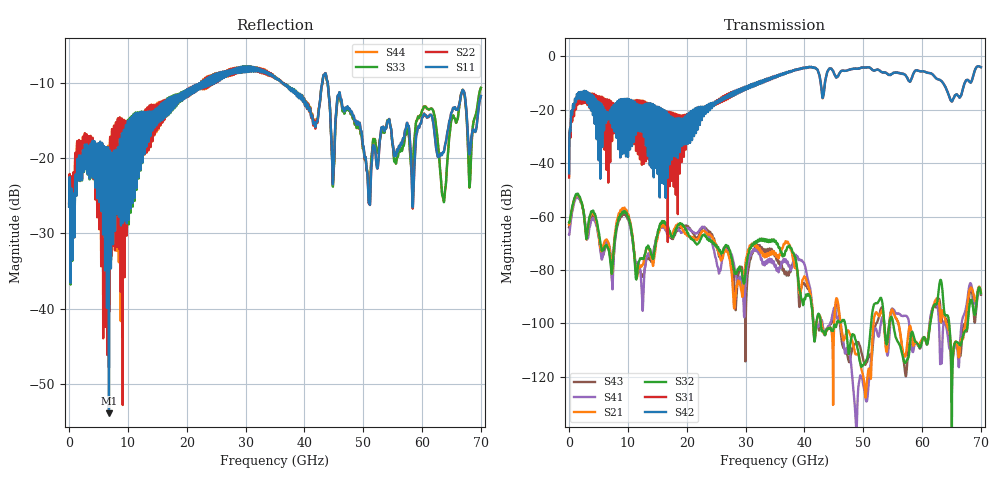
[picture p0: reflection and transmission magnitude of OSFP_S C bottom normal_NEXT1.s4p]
! AWR Design Environment (8415) Mon Jan 07 17:12:19 2019
! Document = 'OSFP Channel_S'
! nPorts: 4, nXvals: 7001
# HZ S DB R 50
!Freq DBS11 AngS11 DBS12 AngS12 DBS13 AngS13 DBS14 AngS14
!	DBS21 AngS21 DBS22 AngS22 DBS23 AngS23 DBS24 AngS24
!	DBS31 AngS31 DBS32 AngS32 DBS33 AngS33 DBS34 AngS34
!	DBS41 AngS41 DBS42 AngS42 DBS43 AngS43 DBS44 AngS44
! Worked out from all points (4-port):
!   7000 points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, 10 MHz to 70 GHz, reference 50 ohm
!   strongest paths, dB at 10 MHz, 17.51 GHz, 35.01 GHz, 52.51 GHz, 70 GHz:
!     S42: -43.8, -27.8, -7.4, -4.9, -4.0
!     S31: -45.4, -27.5, -7.4, -4.9, -4.0
!     S32: -62.3, -67.3, -69.3, -92.1, -88.7
!     S21: -63.1, -66.5, -74.1, -96.7, -88.4
!     S41: -66.8, -66.4, -78.5, -104.6, -88.9
!     S43: -64.1, -67.9, -74.7, -98.7, -89.3
!   lowest |S11| = -53.9 dB at 6.78 GHz (marker M1), VSWR 1.00, Z = 50.1 - j0.161 ohm
!   |S11| at or under -10 dB: start of sweep to 22.43 GHz; 36.26 GHz to 43.05 GHz (6.791 GHz wide, 17.1 % of centre); 43.96 GHz to end of sweep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
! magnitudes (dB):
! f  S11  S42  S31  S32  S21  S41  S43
! 10 MHz  -26.5  -43.8  -45.4  -62.3  -63.1  -66.8  -64.1
! 1.62 GHz  -21.3  -13.4  -15.0  -52.1  -52.4  -53.2  -52.7
! 6.78 GHz  -53.9  -22.4  -17.1  -72.8  -70.6  -70.4  -72.6
! 9.39 GHz  -17.7  -27.8  -23.8  -57.9  -56.7  -57.3  -58.8
! 11.61 GHz  -14.5  -20.7  -18.0  -80.5  -82.0  -77.6  -81.5
! 15.91 GHz  -14.5  -19.8  -20.3  -62.0  -63.3  -63.7  -62.6
! 70 GHz  -11.8  -4.0  -4.0  -88.7  -88.4  -88.9  -89.3
